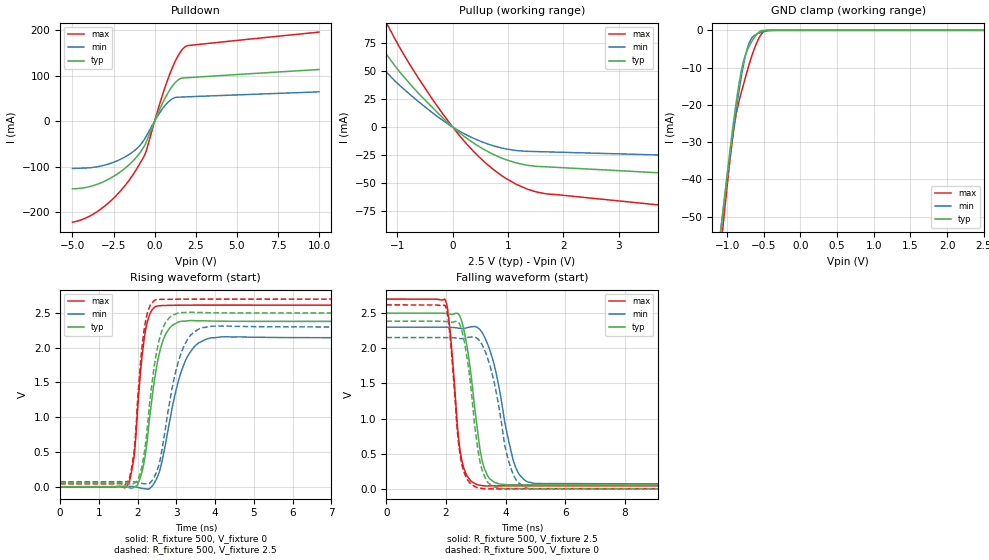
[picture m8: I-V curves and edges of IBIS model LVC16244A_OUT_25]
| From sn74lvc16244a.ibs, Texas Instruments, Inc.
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[Model]   LVC16244A_OUT_25
Model_type  3-state
Enable   Active-Low
Vref =   0
Rref =   500
Cref =   30p
Vmeas =   1.25
| variable   typ   min   max
C_comp   4.83pF   4.40pF   6.03pF
| C_pullup   6.00pF   3.90pF   9.12pF
| C_pulldown   7.52pF   5.42pF   9.58pF
| C_tri-state   4.83pF   4.40pF   6.03pF
[Temperature Range]   40   100   -40
| Ambient temperature   25   85   -40
[Voltage range]   2.5   2.3   2.7
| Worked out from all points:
|   slope of the pulldown table from 0 to 0.375 V, typ, clamps not added: 11.9 ohm
|   slope of the pullup table from 0 to 0.375 V, typ, clamps not added: 26.5 ohm
|   GND clamp passes 1 mA (typ) near -0.59 V on its own axis
|   rising waveform, R_fixture 500, V_fixture 0: 20-80 % time 351ps typ, 512ps min, 236ps max; typ from 0 V to 2.38 V
|   falling waveform, R_fixture 500, V_fixture 2.5: 20-80 % time 435ps typ, 634ps min, 311ps max; typ from 2.5 V to 0.055 V
|   rising waveform, R_fixture 500, V_fixture 2.5: 20-80 % time 330ps typ, 457ps min, 226ps max; typ from 0.055 V to 2.5 V
|   falling waveform, R_fixture 500, V_fixture 0: 20-80 % time 411ps typ, 584ps min, 306ps max; typ from 2.38 V to 0 V
[GND Clamp]
| LVC16244A_OUT_25
|   Voltage   I(typ)   I(min)   I(max)
-5V       -855.7mA   -797.6mA   -953.2mA
-1.09V    -54.36mA   -53.97mA   -59.22mA
-1.06V    -49.06mA   -49.09mA   -53.29mA
-955mV    -31.29mA   -32.66mA   -33.81mA
-900mV    -22.75mA   -24.6mA    -25.4mA
-840mV    -14.58mA   -16.51mA   -19.19mA
-790mV    -9.382mA   -10.63mA   -15.45mA
-730mV    -5.543mA   -5.229mA   -11.2mA
-675mV    -3.361mA   -2.41mA    -7.57mA
-570mV    -549.4uA   -770.8uA   -2.257mA
-490mV    -16.56uA   -280.7uA   -181.4uA
2.5V      9.148pA    37.98nA    -17.36pA
[Pulldown]
| LVC16244A_OUT_25
|   Voltage   I(typ)   I(min)   I(max)
-5V       -148.4mA   -103.9mA   -221.8mA
-4.05V    -144.6mA   -102.7mA   -210.3mA
-3.075V   -132.4mA   -96.92mA   -187.6mA
-2.11V    -112mA     -84.37mA   -154.5mA
-1.27V    -85.53mA   -65.87mA   -114.9mA
-850mV    -67.03mA   -51.33mA   -89.83mA
-540mV    -48.37mA   -34.68mA   -68.09mA
230mV     19.76mA    13.93mA    28.68mA
750mV     58.22mA    39.1mA     86.73mA
1.33V     87.32mA    52.22mA    137mA
1.83V     94.73mA    52.98mA    162.4mA
10V       113.2mA    64.1mA     195.3mA
[Pullup]
| LVC16244A_OUT_25
|   Voltage   I(typ)   I(min)   I(max)
-5V       107mA      39.78mA    366.9mA
-3.895V   252mA      53.48mA    373.6mA
-3.68V    242.4mA    66.07mA    353.2mA
-3.58V    236.9mA    97.7mA     343.4mA
-1.875V   115.8mA    88.65mA    164.7mA
-1.47V    84.95mA    64.9mA     120.5mA
-1.2V     65.32mA    49.39mA    93.48mA
-395mV    18.99mA    13.91mA    27.01mA
320mV     -12.34mA   -8.718mA   -18.78mA
965mV     -29.2mA    -19.52mA   -46.04mA
1.515V    -35.13mA   -21.87mA   -58.07mA
10V       -57.52mA   -33.56mA   -101.4mA
[Ramp]
| LVC16244A_OUT_25
| variable   typ   min   max
dV/dt_r   1.45/3.57E-10   1.31/5.25E-10   1.58/2.41E-10
dV/dt_f   1.47/4.42E-10   1.34/6.51E-10   1.60/3.20E-10
R_load = 500
[Rising Waveform]
| LVC16244A_OUT_25
R_fixture =   500
C_fixture =   0
L_fixture =   0
V_fixture =   0
V_fixture_min = 0
V_fixture_max = 0
|   Time   V(typ)   V(min)   V(max)
0s        140pV      4.165nV    5.164nV
1.77ns    -10.13mV   4.032mV    53.52mV
1.91ns    -7.338mV   1.367mV    445mV
2.08ns    150.2mV    -20.79mV   1.691V
2.195ns   445.8mV    -29.84mV   2.221V
2.54ns    1.869V     182.8mV    2.603V
2.82ns    2.28V      925mV      2.61V
3.245ns   2.386V     1.827V     2.613V
4.16ns    2.382V     2.156V     2.614V
50ns      2.379V     2.145V     2.614V
[Falling Waveform]
| LVC16244A_OUT_25
R_fixture =   500
C_fixture =   0
L_fixture =   0
V_fixture =   2.5
V_fixture_min = 2.3
V_fixture_max = 2.7
|   Time   V(typ)   V(min)   V(max)
0s        2.5V       2.3V       2.7V
1.985ns   2.495V     2.3V       2.68V
2.14ns    2.484V     2.298V     2.231V
2.44ns    2.475V     2.285V     653.5mV
2.705ns   2.022V     2.292V     184.9mV
3.26ns    322.7mV    2.187V     42.52mV
3.63ns    90.28mV    1.739V     40.18mV
4.29ns    57.71mV    355.4mV    41.52mV
4.98ns    55.61mV    75.76mV    41.56mV
50ns      55.34mV    71.05mV    41.67mV
[Rising Waveform]
| LVC16244A_OUT_25
R_fixture =   500
C_fixture =   0
L_fixture =   0
V_fixture =   2.5
V_fixture_min = 2.3
V_fixture_max = 2.7
|   Time   V(typ)   V(min)   V(max)
0s        55.31mV    70.97mV    41.66mV
1.77ns    45.06mV    74.32mV    97.9mV
1.91ns    50.27mV    71.46mV    516.2mV
2.075ns   211.2mV    50.43mV    1.795V
2.185ns   540.9mV    43.93mV    2.319V
2.525ns   2.038V     272mV      2.695V
2.74ns    2.378V     925.5mV    2.696V
3.14ns    2.506V     1.951V     2.699V
3.93ns    2.503V     2.312V     2.7V
50ns      2.5V       2.3V       2.7V
[Falling Waveform]
| LVC16244A_OUT_25
R_fixture =   500
C_fixture =   0
L_fixture =   0
V_fixture =   0
V_fixture_min = 0
V_fixture_max = 0
|   Time   V(typ)   V(min)   V(max)
0s        2.385V     2.152V     2.617V
1.975ns   2.381V     2.152V     2.606V
2.13ns    2.371V     2.151V     2.192V
2.43ns    2.362V     2.141V     613.5mV
2.7ns     1.879V     2.15V      143.2mV
3.04ns    645mV      2.141V     17.17mV
3.26ns    207.9mV    2.008V     410.8uV
4.145ns   -421.2uV   331mV      -113.6uV
4.765ns   483.1uV    2.866mV    -66.43uV
50ns      28.5uV     83.43uV    10.59uV
